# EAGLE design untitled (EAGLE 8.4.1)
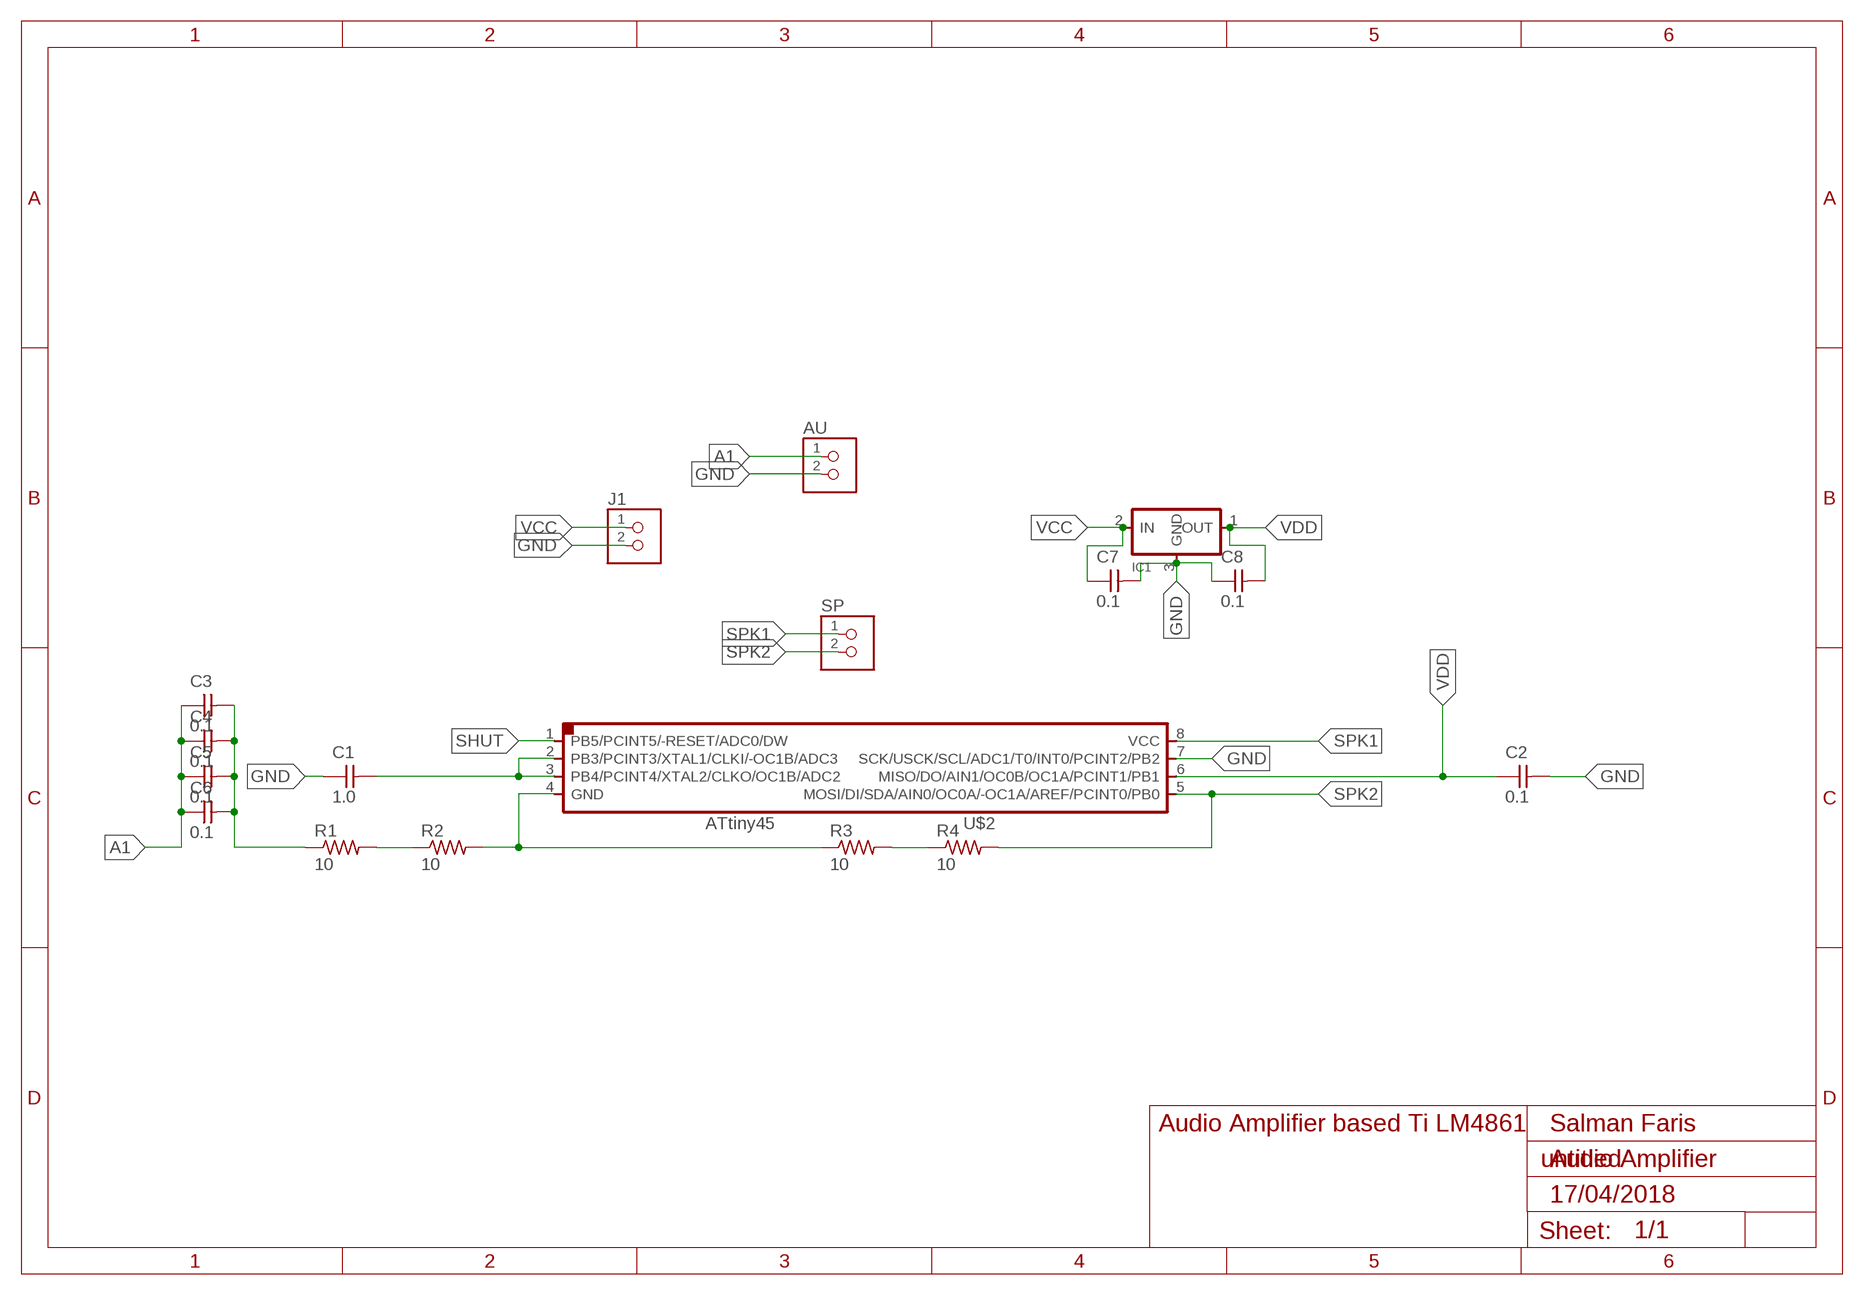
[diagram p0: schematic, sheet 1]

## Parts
AU  TERM-1X02-ADAFRUIT  [3.5MMTERM]
C1  1.0  CAP-UNPOLARIZEDFAB  [C1206FAB]
C2  0.1  CAP-UNPOLARIZEDFAB  [C1206FAB]
C3  0.1  CAP-UNPOLARIZEDFAB  [C1206FAB]
C4  0.1  CAP-UNPOLARIZEDFAB  [C1206FAB]
C5  0.1  CAP-UNPOLARIZEDFAB  [C1206FAB]
C6  0.1  CAP-UNPOLARIZEDFAB  [C1206FAB]
C7  0.1  CAP-UNPOLARIZEDFAB  [C1206FAB]
C8  0.1  CAP-UNPOLARIZEDFAB  [C1206FAB]
IC1  REGULATORSOT23  [SOT23]
J1  TERM-1X02-ADAFRUIT  [3.5MMTERM]
R1  10  RES-US1206FAB  [R1206FAB]
R2  10  RES-US1206FAB  [R1206FAB]
R3  10  RES-US1206FAB  [R1206FAB]
R4  10  RES-US1206FAB  [R1206FAB]
SP  TERM-1X02-ADAFRUIT  [3.5MMTERM]
U$2  ATTINY45SI  [SOIC8]

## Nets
A1: AU.1 C3.1 C4.1 C5.1 C6.1
BYPASS: C1.2 U$2.2(PB3/PCINT3/XTAL1/CLKI/-OC1B/ADC3) U$2.3(PB4/PCINT4/XTAL2/CLKO/OC1B/ADC2)
GND: AU.2 C1.1 C2.2 C7.2 C8.1 IC1.3(GND) J1.2 U$2.7(SCK/USCK/SCL/ADC1/T0/INT0/PCINT2/PB2)
N$1: R2.2 R3.1 U$2.4(GND)
N$13: C3.2 C4.2 C5.2 C6.2 R1.1
N$15: R1.2 R2.1
N$17: R3.2 R4.1
SHUT: U$2.1(PB5/PCINT5/-RESET/ADC0/DW)
SPK1: SP.1 U$2.8(VCC)
SPK2: R4.2 SP.2 U$2.5(MOSI/DI/SDA/AIN0/OC0A/-OC1A/AREF/PCINT0/PB0)
VCC: C7.1 IC1.2(IN) J1.1
VDD: C2.1 C8.2 IC1.1(OUT) U$2.6(MISO/DO/AIN1/OC0B/OC1A/PCINT1/PB1)

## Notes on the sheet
- Audio Amplifier based Ti LM4861 | Salman Faris
- Audio Amplifier
- 17/04/2018

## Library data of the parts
AU J1 SP = fab:TERM-1X02: 3.5mm terminal block, 2 positions ED555-2DS as found in the fablab inventory.
C1-C8 = fab:CAP-UNPOLARIZED
IC1 = fab:REGULATOR
R1-R4 = fab:RES-US: Resistor (US Symbol)
U$2 = fab:ATTINY45

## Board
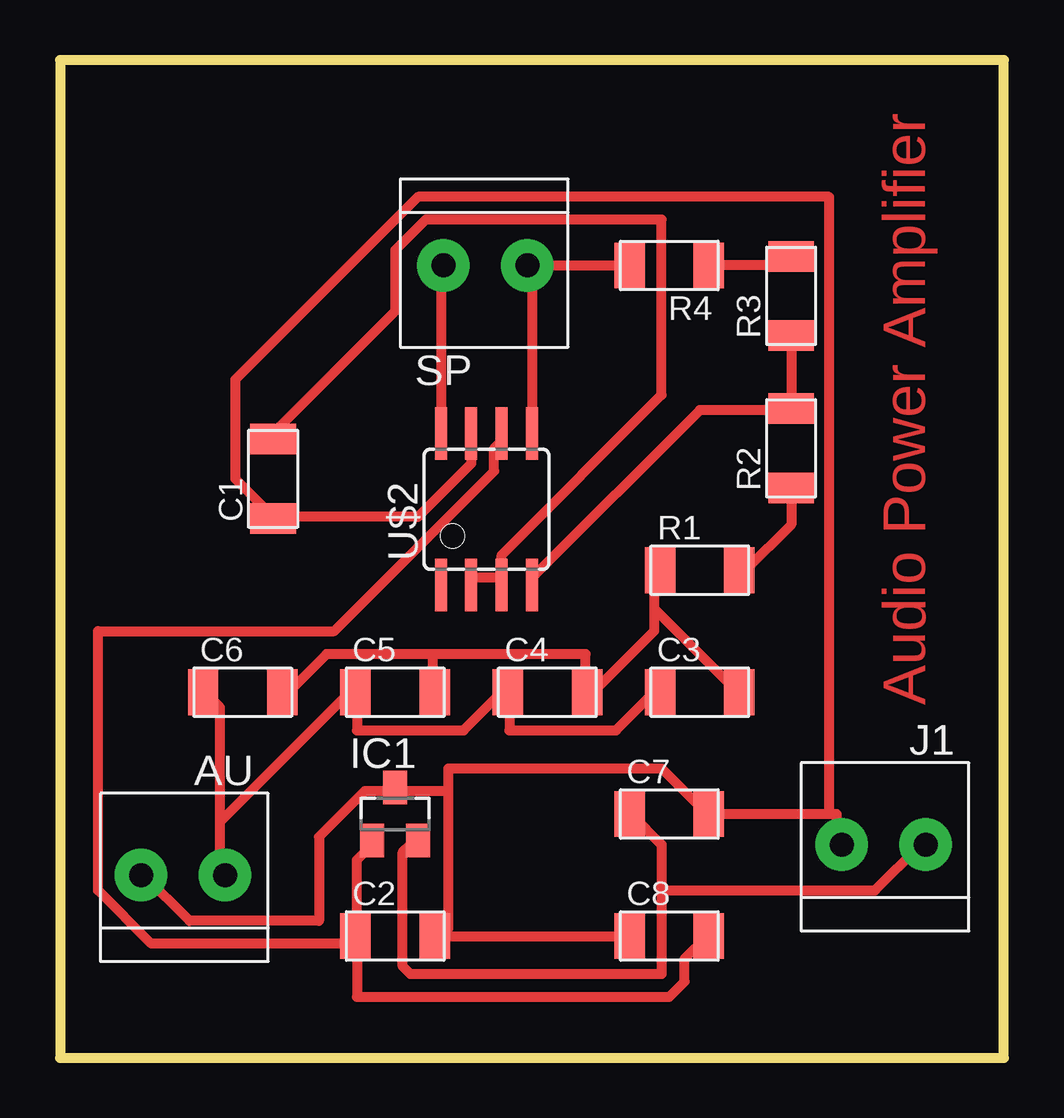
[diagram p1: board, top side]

Size 39.35 x 41.58 mm. Coordinates in mm from the lower left corner, seen from the top.
Outline: 0,0 39.35,0 39.35,41.58 0,41.58 0,0
Copper layers (1*16): Top 0.035mm / dielectric 1.5mm / Bottom 0.035mm
Design rules "default *": minimum track width 16mil, minimum drill 0.35mm, track to track 16mil, track to pad 16mil, pad to pad 16mil, via to via 16mil, smd to smd 16mil, copper to edge 16mil, drill to drill 16mil, minimum pad ring 10mil, minimum via ring 8mil, stop-mask expansion 4mil, vias tented up to drill 0mil, thermal gap 10mil

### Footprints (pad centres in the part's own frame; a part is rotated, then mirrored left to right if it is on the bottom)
3.5MMTERM = drill 1 pad 2.184: 1 1.8,0; 2 -1.7,0
C1206FAB = smd 1.27 x 1.905: 1 -1.651,0; 2 1.651,0
SOT23 = smd 1 x 1.4: 1 -0.95,-1.1; 2 0.95,-1.1; 3 0,1.1
R1206FAB = smd 1.27 x 1.905: 1 -1.651,0; 2 1.651,0
SOIC8 = smd 0.5 x 2.2: 1 -1.905,-3.154; 2 -0.645,-3.154; 3 0.625,-3.154; 4 1.895,-3.154; 5 1.905,3.154; 6 0.635,3.154; 7 -0.635,3.154; 8 -1.905,3.154

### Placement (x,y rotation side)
AU  5.08,7.62 0 top
C1  8.89,24.13 90 top
C2  13.97,5.08 0 top
C3  26.67,15.24 0 top
C4  20.32,15.24 0 top
C5  13.97,15.24 0 top
C6  7.62,15.24 0 top
C7  25.4,10.16 0 top
C8  25.4,5.08 0 top
IC1  13.97,10.16 0 top
J1  34.29,8.89 0 top
R1  26.67,20.32 0 top
R2  30.48,25.4 90 top
R3  30.48,31.75 90 top
R4  25.4,33.02 180 top
SP  17.78,33.02 180 top
U$2  17.78,22.86 0 top

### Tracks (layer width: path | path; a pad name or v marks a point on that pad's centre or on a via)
A1
  Top 0.406: 6.67,9.84 6.67,7.62 AU.1 | 6.67,9.84 6.67,14.61 6.03,15.24 C6.1 | 6.67,9.84 12.06,15.24 C5.1 12.38,15.24 12.38,13.65 16.83,13.65 18.42,15.24 C4.1 18.73,15.24 18.73,13.65 23.18,13.65 24.77,15.24 C3.1
BYPASS
  Top 0.406: 18.42,20 18.42,20.95 25.08,27.62 25.08,34.92 15.24,34.92 13.97,33.66 13.97,31.11 8.89,26.04 C1.2 | 18.42,20 17.14,20 U$2.2 | 18.42,20 U$2.3
GND
  Top 0.406: 8.89,22.54 14.92,22.54 17.14,24.77 U$2.7 | 32.07,10.16 32.38,10.16 32.38,8.89 J1.2 | 32.07,10.16 C7.2 26.99,10.16 25.08,12.06 16.19,12.06 16.19,11.11 | 16.19,11.11 13.97,11.11 | 16.19,11.11 16.19,5.4 15.87,5.08 | 15.87,5.08 C8.1 | 15.87,5.08 C2.2 | 13.97,11.11 12.7,11.11 10.79,9.21 10.79,5.71 5.4,5.71 3.49,7.62 AU.2 | 13.97,11.11 IC1.3 | 8.89,22.54 7.3,24.13 7.3,28.26 14.92,35.88 32.07,35.88 32.07,10.16 | 8.89,22.54 C1.1
N$1
  Top 0.406: R3.1 R2.2 30.48,26.99 26.67,26.99 19.69,20 U$2.4
N$13
  Top 0.406: 15.56,16.83 11.11,16.83 9.53,15.24 C6.2 | 15.56,16.83 15.56,15.24 C5.2 | 24.77,18.73 24.77,20.32 R1.1 | 24.77,18.73 24.77,17.78 22.23,15.24 C4.2 21.91,15.24 21.91,16.83 15.56,16.83 | 24.77,18.73 28.26,15.24 C3.2
N$15
  Top 0.406: R2.1 30.48,22.23 28.57,20.32 R1.2
N$17
  Top 0.406: R4.1 30.48,33.02 R3.2
SPK1
  Top 0.406: U$2.8 15.87,33.02 SP.1
SPK2
  Top 0.406: 19.69,33.02 R4.2 | 19.69,33.02 U$2.5 | 19.69,33.02 SP.2
VCC
  Top 0.406: 25.08,6.99 25.08,8.89 23.81,10.16 C7.1 | 25.08,6.99 25.08,3.49 14.6,3.49 14.29,3.81 14.29,8.57 14.6,8.89 IC1.2 | 25.08,6.99 33.97,6.99 35.88,8.89 J1.1
VDD
  Top 0.406: 12.38,5.08 12.38,8.26 13.02,8.89 IC1.1 | 12.38,5.08 12.38,2.54 25.4,2.54 26.04,3.17 26.04,4.13 26.99,5.08 C8.2 | 12.38,5.08 C2.1 12.06,5.08 12.06,4.76 3.81,4.76 1.59,6.99 1.59,17.78 11.43,17.78 18.1,24.45 18.1,25.4 18.42,25.72 U$2.6

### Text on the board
Top: Audio Power Amplifier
